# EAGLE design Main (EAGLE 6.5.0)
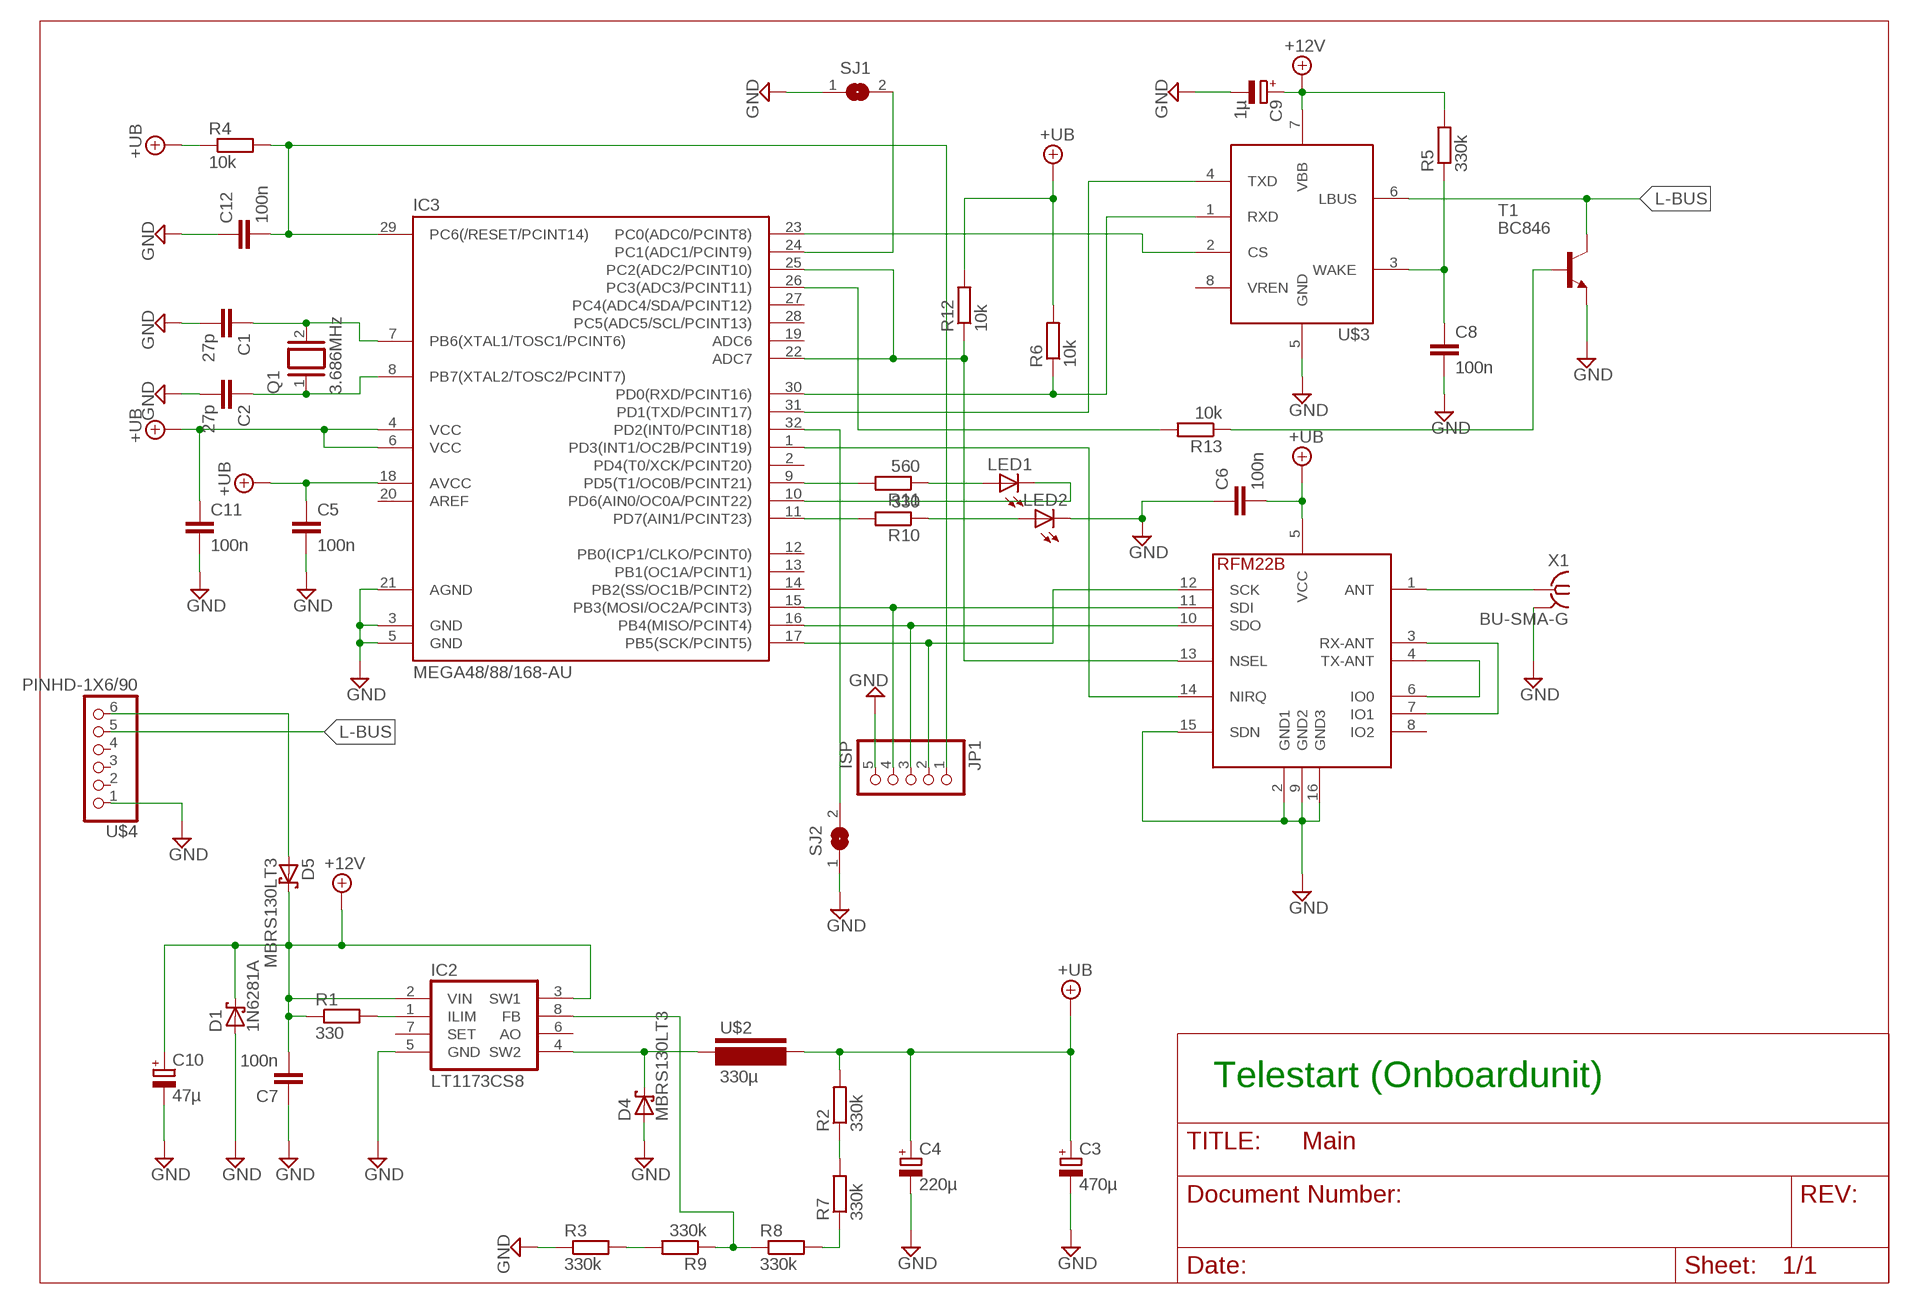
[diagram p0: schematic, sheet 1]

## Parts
C1  27p  C-EUC0603  [C0603]
C2  27p  C-EUC0603  [C0603]
C3  470µ  CPOL-EUF  [PANASONIC_F]
C4  220µ  CPOL-EUUD-6,3X7,7  [UD-6,3X7,7_NICHICON]
C5  100n  C-EUC0805  [C0805]
C6  100n  C-EUC0805  [C0805]
C7  100n  C-EUC0805  [C0805]
C8  100n  C-EUC0805  [C0805]
C9  1µ  CPOL-EUCT3528  [CT3528]
C10  47µ  CPOL-EUF  [PANASONIC_F]
C11  100n  C-EUC0805  [C0805]
C12  100n  C-EUC0805  [C0805]
D1  1N6281A  1N6267A  [C4111-15]
D4  MBRS130LT3  [SMB]
D5  MBRS130LT3  [SMB]
IC2  LT1173CS8  [SO08]
IC3  MEGA48/88/168-AU  [TQFP32-08]
JP1  ISP  PINHD-1X5  [1X05]
LED1  LED3MM  [LED3MM]
LED2  LED3MM  [LED3MM]
Q1  3.686MHz  XTAL/S  [QS]
R1  330  R-EU_M0805  [M0805]
R2  330k  R-EU_M1206  [M1206]
R3  330k  R-EU_M1206  [M1206]
R4  10k  R-EU_M1206  [M1206]
R5  330k  R-EU_M1206  [M1206]
R6  10k  R-EU_M1206  [M1206]
R7  330k  R-EU_M1206  [M1206]
R8  330k  R-EU_M1206  [M1206]
R9  330k  R-EU_M1206  [M1206]
R10  330  R-EU_M1206  [M1206]
R11  560  R-EU_M1206  [M1206]
R12  10k  R-EU_M0805  [M0805]
R13  10k  R-EU_M1206  [M1206]
SJ1  SJ  [SJ]
SJ2  SJ  [SJ]
T1  BC846  [SOT23]
U$1  RFM22B_SMD  [RFM_16PIN_SMD]
U$2  330µ  L-PISM  [PISM]
U$3  MCP2003SIOC  [SO-08]
U$4  PINHD-1X6/90  [1X06/90]
X1  BU-SMA-G  [BU-SMA-G]

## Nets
$N100: D5.A U$4.6
+12V: C7.2 C9.+ C10.+ D1.C D5.C IC2.2(VIN) IC2.3(SW1) R1.1 R5.2 U$3.7(VBB)
+UB: C3.+ C4.+ C5.1 C6.2 C11.1 IC3.4(VCC) IC3.6(VCC) IC3.18(AVCC) R2.2 R4.1 R6.2 R12.2 U$1.5(VCC) U$2.P$2
GND: C1.2 C2.2 C3.- C4.- C5.2 C6.1 C7.1 C8.2 C9.- C10.- C11.2 C12.1 D1.A D4.A IC2.5(GND) IC3.3(GND) IC3.5(GND) IC3.21(AGND) JP1.5 LED2.K(C) R3.1 SJ1.1 SJ2.1 T1.2(E) U$1.2(GND1) U$1.9(GND2) U$1.15(SDN) U$1.16(GND3) U$3.5(GND) U$4.1 X1.2 X1.3 X1.4 X1.5
L-BUS: T1.3(C) U$3.6(LBUS) U$4.5
N$1: U$1.4(TX-ANT) U$1.6(IO0)
N$2: U$1.3(RX-ANT) U$1.7(IO1)
N$3: IC3.17(PB5(SCK/PCINT5)) JP1.2 U$1.12(SCK)
N$4: IC3.16(PB4(MISO/PCINT4)) JP1.3 U$1.10(SDO)
N$5: IC3.15(PB3(MOSI/OC2A/PCINT3)) JP1.4 U$1.11(SDI)
N$6: IC3.1(PD3(INT1/OC2B/PCINT19)) U$1.14(NIRQ)
N$7: IC3.22(ADC7) IC3.25(PC2(ADC2/PCINT10)) R12.1 U$1.13(NSEL)
N$8: C12.2 IC3.29(PC6(/RESET/PCINT14)) JP1.1 R4.2
N$9: C1.1 IC3.7(PB6(XTAL1/TOSC1/PCINT6)) Q1.2
N$10: IC3.31(PD1(TXD/PCINT17)) U$3.4(TXD)
N$11: C2.1 IC3.8(PB7(XTAL2/TOSC2/PCINT7)) Q1.1
N$12: IC2.1(ILIM) R1.2
N$13: U$1.1(ANT) X1.1
N$14: IC3.30(PD0(RXD/PCINT16)) R6.1 U$3.1(RXD)
N$15: D4.C IC2.4(SW2) U$2.P$1
N$17: R3.2 R9.2
N$18: C8.1 R5.1 U$3.3(WAKE)
N$19: IC3.23(PC0(ADC0/PCINT8)) U$3.2(CS)
N$20: IC3.32(PD2(INT0/PCINT18)) SJ2.2
N$22: IC2.8(FB) R8.1 R9.1
N$23: R7.1 R8.2
N$24: R2.1 R7.2
N$25: IC3.24(PC1(ADC1/PCINT9)) SJ1.2
N$26: IC3.9(PD5(T1/OC0B/PCINT21)) R11.2
N$27: IC3.10(PD6(AIN0/OC0A/PCINT22)) LED1.K(C)
N$28: LED1.A R11.1
N$29: IC3.11(PD7(AIN1/PCINT23)) R10.2
N$30: LED2.A R10.1
N$35: IC3.26(PC3(ADC3/PCINT11)) R13.2
N$36: R13.1 T1.1(B)
Unconnected: IC2.6(AO) IC2.7(SET) IC3.2(PD4(T0/XCK/PCINT20)) IC3.12(PB0(ICP1/CLKO/PCINT0)) IC3.13(PB1(OC1A/PCINT1)) IC3.14(PB2(SS/OC1B/PCINT2)) IC3.19(ADC6) IC3.20(AREF) IC3.27(PC4(ADC4/SDA/PCINT12)) IC3.28(PC5(ADC5/SCL/PCINT13)) U$1.8(IO2) U$3.8(VREN) U$4.2 U$4.3 U$4.4

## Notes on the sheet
- Telestart (Onboardunit)

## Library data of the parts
C1 C2 C5-C8 C11 C12 = rcl:C-EU: CAPACITOR, European symbol
C3 C4 C9 C10 = rcl:CPOL-EU: POLARIZED CAPACITOR, European symbol
D1 = diode:1N6267A: DIODE
D4 D5 = diode:MBRS130LT3: Schottky Power Rectifier
IC2 = linear-technology-3:LT1173*: Micropower DC/DC Converter Adjustable and Fixed 5V, 12V
IC3 = avr-4:MEGA48/88/168
JP1 = pinhead:PINHD-1X5: PIN HEADER
LED1 LED2 = led:LED: LED
Q1 = special:XTAL/S: CRYSTAL
R1-R13 = rcl:R-EU_: RESISTOR, European symbol
SJ1 SJ2 = jumper:SJ: SMD solder JUMPER
T1 = transistor:BC846: NPN TRANSISTOR
U$1 = rfm:RFM22B_SMD
U$2 = L-PISR:L-PISM
U$3 = microchip_can-lin:MCP2003: LIN J2602 Transceiver
U$4 = pinhead:PINHD-1X6/90
X1 = con-coax:BU-SMA-G: FEMALE SMA CONNECTOR; OC_FARNELL: unknown; OC_NEWARK: unknown

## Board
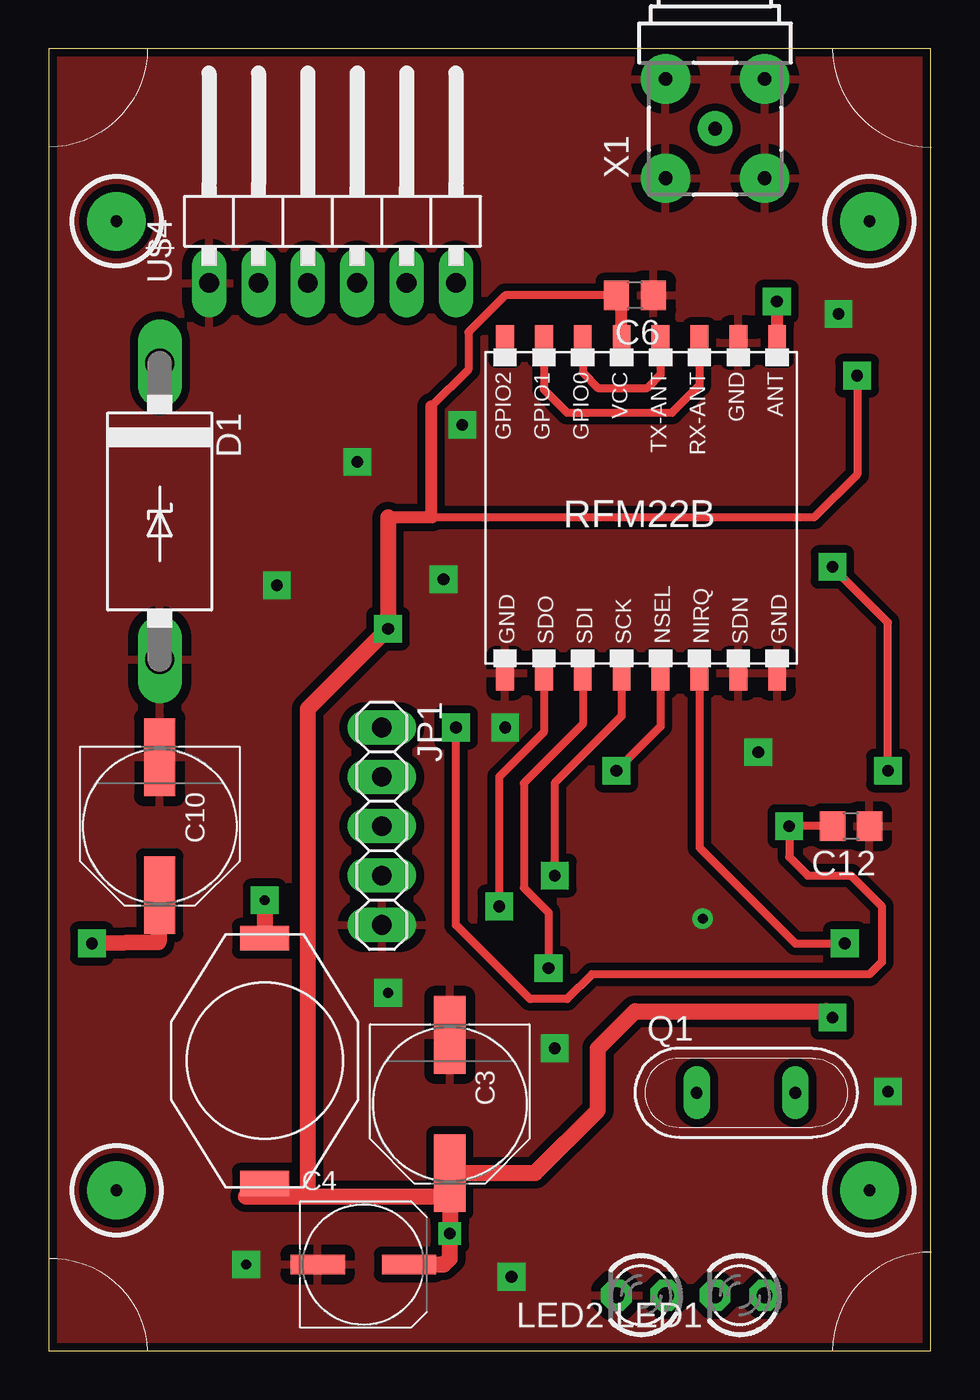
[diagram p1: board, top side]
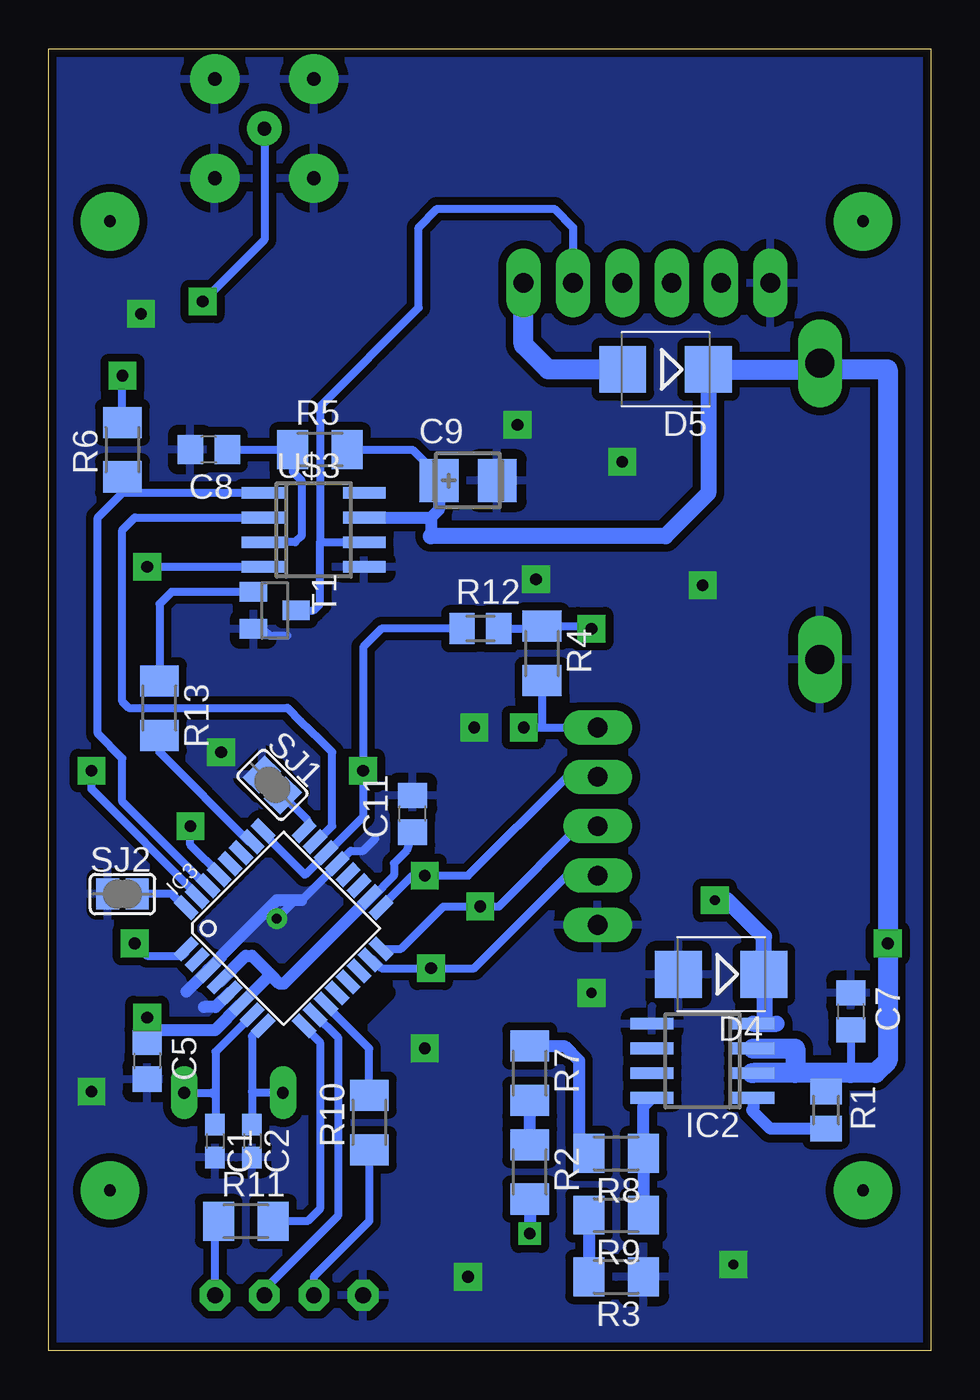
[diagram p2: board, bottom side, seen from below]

Size 45.39 x 66.98 mm. Coordinates in mm from the lower left corner, seen from the top.
Outline: 0,0 45.39,0 45.39,66.98 0,66.98 0,0
Copper layers (1*16): Top 0.035mm / dielectric 1.5mm / Bottom 0.035mm
Design rules "default *": minimum track width 10mil, minimum drill 60mil, track to track 8mil, track to pad 8mil, pad to pad 8mil, via to via 8mil, smd to smd 8mil, copper to edge 1mil, drill to drill 8mil, minimum pad ring 15mil, minimum via ring 11mil, stop-mask expansion 4mil, vias tented up to drill 0mil, thermal gap 20mil
bRestrict: area 27.9,16.8 to 30.2,19.1

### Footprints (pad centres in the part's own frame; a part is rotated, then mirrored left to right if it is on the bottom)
C0603 = smd 1.1 x 1: 1 -0.85,0; 2 0.85,0
PANASONIC_F = smd 4 x 1.6: + 3.55,0; - -3.55,0
UD-6,3X7,7_NICHICON = smd 2.8 x 1: + 2.35,0; - -2.35,0
C0805 = smd 1.3 x 1.5: 1 -0.95,0; 2 0.95,0
CT3528 = smd 2 x 2.2: + -1.5,0; - 1.5,0
C4111-15 = drill 1.499 long: A 7.62,0; C -7.62,0
SMB = smd 2.4 x 2.4: A 2.2,0; C -2.2,0
SO08 = smd 0.6 x 2.2: 1 -1.905,-2.6; 2 -0.635,-2.6; 3 0.635,-2.6; 4 1.905,-2.6; 5 1.905,2.6; 6 0.635,2.6; 7 -0.635,2.6; 8 -1.905,2.6
TQFP32-08 = smd 1.27 x 0.559: 1 -4.293,2.8; 2 -4.293,2; 3 -4.293,1.2; 4 -4.293,0.4; 5 -4.293,-0.4; 6 -4.293,-1.2; 7 -4.293,-2; 8 -4.293,-2.8; 17 4.293,-2.8; 18 4.293,-2; 19 4.293,-1.2; 20 4.293,-0.4; 21 4.293,0.4; 22 4.293,1.2; 23 4.293,2; 24 4.293,2.8 | smd 0.559 x 1.27: 9 -2.8,-4.293; 10 -2,-4.293; 11 -1.2,-4.293; 12 -0.4,-4.293; 13 0.4,-4.293; 14 1.2,-4.293; 15 2,-4.293; 16 2.8,-4.293; 25 2.8,4.293; 26 2,4.293; 27 1.2,4.293; 28 0.4,4.293; 29 -0.4,4.293; 30 -1.2,4.293; 31 -2,4.293; 32 -2.8,4.293
1X05 = drill 1.016 long: 1 -5.08,0; 2 -2.54,0; 3 0,0; 4 2.54,0; 5 5.08,0
LED3MM = drill 0.813 octagon: A -1.27,0; K 1.27,0
QS = drill 0.61 long: 1 -2.54,0; 2 2.54,0
M0805 = smd 1.3 x 1.6: 1 -0.95,0; 2 0.95,0
M1206 = smd 1.6 x 2: 1 -1.4,0; 2 1.4,0
SJ = smd 1.168 x 1.6: 1 -0.762,0; 2 0.762,0
SOT23 = smd 1 x 1.4: 1 -0.95,-1.1; 2 0.95,-1.1; 3 0,1.1
RFM_16PIN_SMD = smd 1.778 x 0.914: 1 -9,7; 2 -9,5; 3 -9,3; 4 -9,1; 5 -9,-1; 6 -9,-3; 7 -9,-5; 8 -9,-7; 9 8,-7; 10 8,-5; 11 8,-3; 12 8,-1; 13 8,1; 14 8,3; 15 8,5; 16 8,7
PISM = smd 1.27 x 2.54: P$1 -6.3,0; P$2 6.3,0
SO-08 = smd 0.6 x 2.2: 1 -1.905,-2.6; 2 -0.635,-2.6; 3 0.635,-2.6; 4 1.905,-2.6; 5 1.905,2.6; 6 0.635,2.6; 7 -0.635,2.6; 8 -1.905,2.6
1X06/90 = drill 1.016 long: 1 -6.35,-3.81; 2 -3.81,-3.81; 3 -1.27,-3.81; 4 1.27,-3.81; 5 3.81,-3.81; 6 6.35,-3.81
BU-SMA-G = drill 0.7 pad 1.778: 1 0,0 | drill 0.7 pad 2.54: 2 -2.55,2.55; 3 2.55,2.55; 4 2.55,-2.55; 5 -2.55,-2.55

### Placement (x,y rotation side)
C1  36.83,10.79 270 bottom
C2  34.92,10.79 270 bottom
C3  20.64,12.7 270 top
C4  16.19,4.45 0 top
C5  40.32,14.92 270 bottom
C6  30.16,54.29 180 top
C7  4.13,17.46 270 bottom
C8  37.15,46.36 180 bottom
C9  23.81,44.77 0 bottom
C10  5.71,26.99 270 top
C11  26.67,27.62 90 bottom
C12  41.27,26.99 180 top
D1  5.71,43.18 270 top
D4  10.79,19.37 180 bottom
D5  13.65,50.48 180 bottom
IC2  11.75,14.92 90 bottom
IC3  33.3,21.74 45 bottom
JP1  17.14,26.99 270 top
LED1  35.56,2.86 180 top
LED2  30.48,2.86 180 top
Q1  35.88,13.28 0 top
R1  5.4,12.38 270 bottom
R2  20.64,9.21 270 bottom
R3  16.19,3.81 180 bottom
R4  20,35.88 270 bottom
R5  31.43,46.36 0 bottom
R6  41.59,46.36 90 bottom
R7  20.64,14.29 270 bottom
R8  16.19,10.16 180 bottom
R9  16.19,6.98 180 bottom
R10  28.89,11.75 90 bottom
R11  35.24,6.67 0 bottom
R12  23.18,37.15 0 bottom
R13  39.69,33.06 270 bottom
SJ1  33.88,29.12 315 bottom
SJ2  41.59,23.5 0 bottom
T1  33.75,38.09 270 bottom
U$1  30.48,42.86 270 top
U$2  11.11,14.92 270 top
U$3  31.75,42.23 270 bottom
U$4  14.61,58.74 0 top
X1  34.29,62.87 90 top

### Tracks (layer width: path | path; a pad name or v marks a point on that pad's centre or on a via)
$N100
  Bottom 1.016: D5.A 19.68,50.48 20.95,51.75 U$4.6
+12V  (via drill 0.6 pad 1.42)
  Top 0.813: C10.+ 5.66,21.01 v2.22,20.96
  Bottom 0.406: IC2.2 6.99,14.29 5.9,14.29 R1.1 | R5.2 26.67,46.36 25.31,45 C9.+ | C7.2 4.13,14.29
  Bottom 0.61: U$3.7 25.72,42.86 | 25.72,42.86 25.72,41.91 | C9.+ 25.31,43.27 25.72,42.86
  Bottom 0.813: 25.72,41.91 13.65,41.91 11.45,44.11 D5.C
  Bottom 1.016: IC2.3 6.99,15.56 6.99,14.29 | 9.21,14.29 IC2.2 4.13,14.29 2.86,14.29 2.22,14.92 v2.22,20.96 2.22,50.48 5.71,50.48 | D5.C 5.71,50.48 | 5.71,50.48 D1.C
+UB  (via drill 0.6 pad 0.81, 0.6 pad 1.42)
  Top 0.406: v41.59,50.16 41.59,45.08 39.37,42.86 19.73,42.86 | 19.68,48.58 21.59,50.48 21.59,52.39 23.5,54.29 C6.2
  Top 0.61: 17.46,42.86 19.73,42.86 19.68,42.91 19.68,48.58 | U$1.5 29.48,54.02 C6.2
  Top 0.813: 17.46,42.86 v17.46,37.15 13.34,33.02 13.34,7.94 | v40.32,17.15 40.01,17.46 30.16,17.46 28.26,15.56 28.26,12.38 25.02,9.15 C3.+ | 20.64,9.21 C3.+ | C4.+ 20.32,4.44 20.64,4.76 v20.64,6.03 20.64,7.94 | C3.+ 20.64,7.94 | U$2.P$2 10.85,8.62 10.16,7.94 13.34,7.94 | 13.34,7.94 20.64,7.94
  Bottom 0.406: IC3.4 36.58,18.98 | 35.53,17.81 | 35.53,17.81 IC3.6 | IC3.18 28.71,23.36 27.62,24.45 27.62,25.08 26.99,25.72 C11.1 | R6.2 v41.59,50.16 | v17.46,37.15 17.59,37.28 R4.1 20.13,37.15 R12.2
  Bottom 0.61: 35.53,17.81 36.85,16.49 39.7,16.49 v40.32,17.15 | 36.58,18.98 35.24,20.32 34.92,20.32 34.2,19.59 34.2,19.58 33.98,19.36 | 34.29,19.05 IC3.6 | IC3.18 28.85,23.33 33.3,18.88 33.5,18.88 33.98,19.36 | 34.29,19.05 | 34.29,19.05 33.98,19.36 | R2.2 v20.64,6.03
  Bottom 0.813: C5.1 v40.32,17.15
GND  (via drill 0.5, 0.5 pad 1.42, 0.6 pad 1.42)
  Bottom 0.406: IC3.21 30.51,25.06 | 30.51,25.06 29.84,25.72 29.21,25.72 28.57,26.35 | 30.51,25.06 32.38,23.18 | T1.2 34.35,37.14 34,36.78 33.1,36.78 | 33.34,22.54 32.7,23.18
  Bottom 0.61: 32.38,23.18 32.7,23.18 33.66,23.18 36.5,20.33 36.5,20.28 37.18,19.6 IC3.3 37.23,19.55 38.3,18.48 | IC3.5 36.8,17.68 37.4,17.68
  other vias: 21.27,47.62 26.04,15.56 23.5,32.07 11.75,39.37 40.64,53.34 43.18,13.33 36.51,30.8 23.81,3.81 20.32,39.69 15.88,45.72 33.66,22.23 17.46,18.42 10.16,4.45
  pour Bottom (isolate 0.406): -0.64,67.63 46.99,67.63 46.99,-0.95 45.4,-2.54 -0.64,-2.54 -1.27,-1.9 -1.27,66.99
  pour Top (isolate 0.406): -1.59,68.26 46.35,68.26 46.67,67.94 46.67,-0.95 45.09,-2.54 0,-2.54 -0.95,-1.59 -0.95,67.63 -1.27,67.94
L-BUS
  Bottom 0.406: 31.43,41.59 31.43,48.58 26.35,53.66 26.35,57.79 25.4,58.74 19.37,58.74 18.41,57.79 U$4.5 | 31.43,41.59 U$3.6 | T1.3 31.76,38.09 31.43,38.42 31.43,41.59
N$1
  Top 0.406: U$1.6 27.48,50.31 28.26,49.53 30.8,49.53 31.48,50.21 U$1.4
N$2
  Top 0.406: U$1.7 25.48,49.45 26.67,48.26 32.07,48.26 33.48,49.67 U$1.3
N$3  (via drill 0.6 pad 1.42)
  Top 0.406: v26.04,24.45 26.04,29.21 29.48,32.65 U$1.12
  Bottom 0.406: JP1.2 18.73,29.53 23.81,24.45 v26.04,24.45 26.67,24.45 28.28,22.83 IC3.17
N$4  (via drill 0.6 pad 1.42)
  Top 0.406: U$1.10 25.48,31.83 23.18,29.53 v23.18,22.86
  Bottom 0.406: JP1.3 18.1,26.99 22.23,22.86 v23.18,22.86 25.08,22.86 27.26,20.68 IC3.16
N$5  (via drill 0.6 pad 1.42)
  Top 0.406: v25.72,19.69 25.72,22.54 24.45,23.81 24.45,29.21 27.48,32.24 U$1.11
  Bottom 0.406: JP1.4 18.73,24.45 23.5,19.69 v25.72,19.69 28.26,19.69 28.69,20.12 IC3.15
N$6  (via drill 0.6 pad 1.42)
  Top 0.406: U$1.14 33.48,25.89 38.42,20.96 v40.96,20.96
  Bottom 0.406: v40.96,20.96 40.32,20.32 38.52,20.32 38.31,20.52 IC3.1
N$7  (via drill 0.6 pad 1.42)
  Top 0.406: v29.21,29.85 31.48,32.12 U$1.13
  Bottom 0.406: IC3.25 34.35,26.64 32.2,24.48 31.11,25.57 IC3.22 31.06,25.62 29.21,27.47 v29.21,29.85 29.21,36.19 28.26,37.15 R12.1
N$8  (via drill 0.6 pad 1.42)
  Top 0.406: C12.2 v38.1,26.99 38.1,25.4 39.05,24.45 41.27,24.45 42.86,22.86 42.86,20 42.23,19.37 27.94,19.37 26.67,18.1 24.77,18.1 20.95,21.91 v20.95,32.07
  Bottom 0.406: v38.1,26.99 38.1,26.03 36.51,24.45 36.57,24.45 IC3.29 | v20.95,32.07 20,32.07 | 20,32.07 JP1.1 | R4.2 20,32.07
N$9
  Bottom 0.406: IC3.7 34.92,17.26 36.8,15.38 36.8,13.08 | 36.8,13.08 36.8,12.1 37.15,11.75 36.96,11.75 36.8,11.58 36.8,11.61 C1.1 | Q1.2 37,13.28 36.8,13.08
N$10  (via drill 0.6 pad 1.42)
  Top 0.406: v43.18,29.85 43.18,37.47 v40.32,40.32
  Bottom 0.406: v43.18,29.85 43.18,28.89 37.63,23.35 37.74,23.35 IC3.31 | U$3.4 v40.32,40.32
N$11
  Bottom 0.406: 34.92,13.33 34.92,16.19 34.4,16.72 IC3.8 | 34.92,13.33 C2.1 | Q1.1 34.87,13.28 34.92,13.33
N$12
  Bottom 0.61: R1.2 8.26,11.43 9.21,12.38 9.15,12.44 IC2.1
N$13  (via drill 0.6 pad 1.42)
  Top 0.61: U$1.1 37.48,53.96 v37.47,53.97
  Bottom 0.406: v37.47,53.97 34.29,57.15 X1.1
N$14
  Bottom 0.406: U$3.1 41.59,44.13 | 37.22,23.88 37.22,23.89 | 37.22,23.89 IC3.30 | 41.59,44.13 42.86,42.86 42.86,31.75 41.59,30.48 41.59,28.26 37.23,23.89 37.22,23.89 | R6.1 41.59,44.13
N$15  (via drill 0.5 pad 1.42)
  Top 0.813: v11.11,23.18 U$2.P$1
  Bottom 0.813: IC2.4 8.57,16.83 | 8.57,16.83 7.94,16.83 | 8.57,16.83 8.57,19.05 8.89,19.37 D4.C 8.6,21.3 10.48,23.18 v11.11,23.18
N$16  (via drill 0.6 pad 3)
  other vias: 3.49,58.1
N$17
  Bottom 0.61: R9.2 R3.2
N$18
  Bottom 0.406: R5.1 32.83,45.22 32.38,44.77 32.38,41.91 32.7,41.59 U$3.3 | C8.1 R5.1 | R5.1 32.7,46.04
N$19
  Bottom 0.406: IC3.23 31.6,26.19 30.8,26.99 30.8,30.8 31.43,31.43 32.41,32.38 33.1,33.07 41.26,33.07 41.59,33.41 41.59,42.23 40.96,42.86 U$3.2 33.97,42.86
N$20
  Bottom 0.406: IC3.32 38.35,22.79 39.05,23.49 SJ2.2
N$22
  Bottom 0.61: IC2.8 14.79,12.57 R8.1 R9.1
N$23
  Bottom 0.61: R7.1 18.86,15.69 18.1,14.92 18.1,10.66 R8.2
N$24
  Bottom 0.61: R2.1 R7.2
N$25
  Bottom 0.406: SJ1.2 | SJ1.2 32.07,27.3 32.07,26.93 IC3.24
N$26
  Bottom 0.406: IC3.9 32.24,16.69 31.43,15.87 31.43,7.3 32.07,6.67 R11.2
N$27
  Bottom 0.406: LED1.K 34.29,3.18 30.48,6.98 30.48,16.09 IC3.10
N$28
  Bottom 0.406: LED1.A 36.83,6.48 R11.1
N$29
  Bottom 0.406: IC3.11 31.11,17.78 28.89,15.56 R10.2
N$30
  Bottom 0.406: R10.1 28.89,6.67 31.75,3.81 LED2.A
N$35
  Bottom 0.406: IC3.26 35.08,26.19 39.69,30.8 R13.2
N$36
  Bottom 0.406: T1.1 39.07,39.04 39.69,38.42 R13.1
N$37  (via drill 0.6 pad 3)
  other vias: 42.23,58.1
N$38  (via drill 0.6 pad 3)
  other vias: 42.23,8.25
N$39  (via drill 0.6 pad 3)
  other vias: 3.49,8.25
